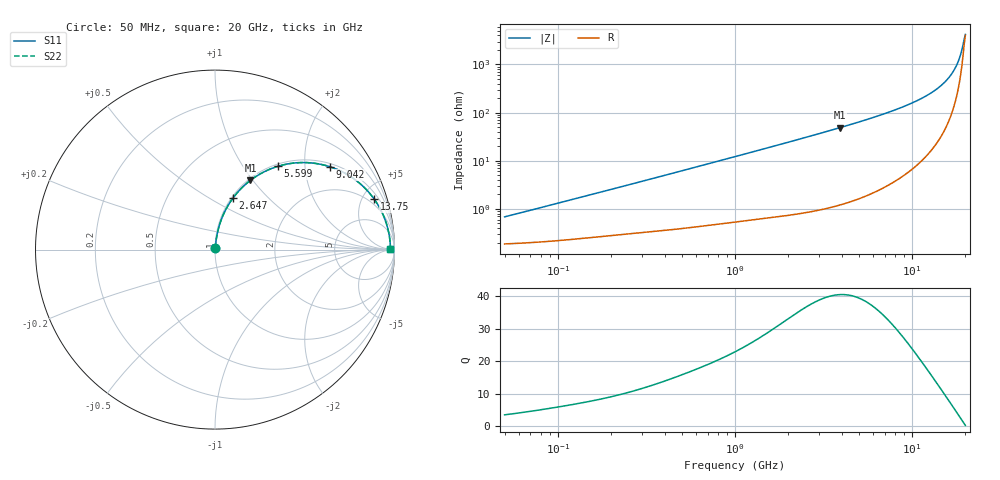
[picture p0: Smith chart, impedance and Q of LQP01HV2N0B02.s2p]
!Murata Part Number: LQP01HV2N0B02
!These Parameters are Measured in Series Mode Connection
!  o--[Z]--o
!Port1  Port2
!  o-------o
!Freq. Start=50[MHz] Stop=20[GHz], 401[Steps]
# Hz S RI R 50
!Freq.(Hz) S11(Real) S11(Imag) S21(Real) S21(Imag) S12(Real) S12(Imag) S22(Real) S22(Imag)
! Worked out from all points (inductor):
!   401 points, 50 MHz to 20 GHz, reference 50 ohm
!   read as one part in series: L = 2.09 nH near 51.52 MHz
!   highest Q = 40.4 at 3.908 GHz (marker M1), where L = 1.98 nH
!   S11 on the Smith chart (normalised r, x): 50 MHz: 1.00, +0.01; 2.647 GHz: 1.02, +0.65; 5.599 GHz: 1.04, +1.45; 9.042 GHz: 1.10, +2.71; 13.75 GHz: 1.46, +6.13; 20 GHz: 82, +21
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5e7  0.00191 0.00656  0.9981 -0.00656  0.9981 -0.00656  0.00191 0.00656
1.364002e8  0.00273 0.0174  0.9973 -0.0174  0.9973 -0.0174  0.00273 0.0174
3.721004e8  0.00557 0.0458  0.9944 -0.0458  0.9944 -0.0458  0.00557 0.0458
1e9  0.0197 0.1187  0.9803 -0.1187  0.9803 -0.1187  0.0197 0.1187
1.740566e9  0.0487 0.1995  0.9513 -0.1995  0.9513 -0.1995  0.0487 0.1995
2.647493e9  0.1009 0.2881  0.8991 -0.2881  0.8991 -0.2881  0.1009 0.2881
2.728004e9  0.1063 0.2953  0.8937 -0.2953  0.8937 -0.2953  0.1063 0.2953
3.908127e9  0.1972 0.3857  0.8028 -0.3857  0.8028 -0.3857  0.1972 0.3857
5.598765e9  0.349 0.4637  0.651 -0.4637  0.651 -0.4637  0.349 0.4637
7.442007e9  0.5147 0.4845  0.4853 -0.4845  0.4853 -0.4845  0.5147 0.4845
9.041845e9  0.642 0.4612  0.358 -0.4612  0.358 -0.4612  0.642 0.4612
1.149051e10  0.7935 0.3798  0.2065 -0.3798  0.2065 -0.3798  0.7935 0.3798
1.375312e10  0.8872 0.281  0.1128 -0.281  0.1128 -0.281  0.8872 0.281
1.482269e10  0.918 0.2318  0.082 -0.2318  0.082 -0.2318  0.918 0.2318
1.573793e10  0.9385 0.1897  0.0615 -0.1897  0.0615 -0.1897  0.9385 0.1897
1.646126e10  0.9511 0.1567  0.0489 -0.1567  0.0489 -0.1567  0.9511 0.1567
1.721783e10  0.9614 0.1228  0.0386 -0.1228  0.0386 -0.1228  0.9614 0.1228
1.774144e10  0.9669 0.0998  0.0331 -0.0998  0.0331 -0.0998  0.9669 0.0998
1.828096e10  0.9712 0.0765  0.0288 -0.0765  0.0288 -0.0765  0.9712 0.0765
1.88369e10  0.9744 0.053  0.0256 -0.053  0.0256 -0.053  0.9744 0.053
1.970266e10  0.9771 0.0175  0.0229 -0.0175  0.0229 -0.0175  0.9771 0.0175
2e10  0.9774 0.00562  0.0226 -0.00562  0.0226 -0.00562  0.9774 0.00562
